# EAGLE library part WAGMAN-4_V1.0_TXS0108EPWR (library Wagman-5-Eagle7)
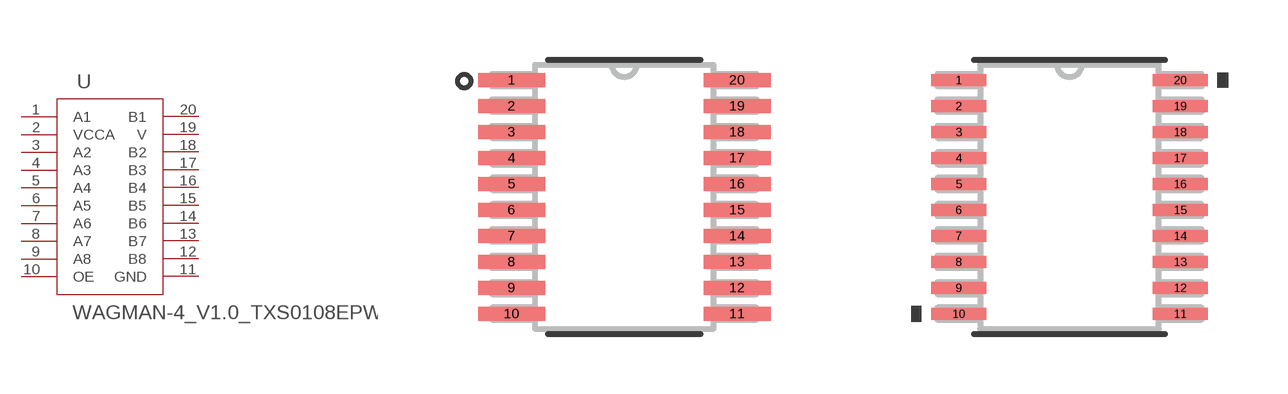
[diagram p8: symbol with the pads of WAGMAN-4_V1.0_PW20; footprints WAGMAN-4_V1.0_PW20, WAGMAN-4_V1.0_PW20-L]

Designator prefix U

## WAGMAN-4_V1.0_TXS0108EPWR (MANUFACTURER_PART_NUMBER: TXS0108EPWR; VENDOR: Texas Instruments)  [WAGMAN-4_V1.0_PW20]
1  A1
2  VCCA  pwr
3  A2
4  A3
5  A4
6  A5
7  A6
8  A7
9  A8
10  OE  out
11  GND  pwr
12  B8
13  B7
14  B6
15  B5
16  B4
17  B3
18  B2
19  V  pwr
20  B1

## WAGMAN-4_V1.0_TXS0108EPWRPW20-L (MANUFACTURER_PART_NUMBER: TXS0108EPWR; VENDOR: Texas Instruments)  [WAGMAN-4_V1.0_PW20-L]
Pads as for WAGMAN-4_V1.0_PW20

## WAGMAN-4_V1.0_TXS0108EPWRPW20-M (MANUFACTURER_PART_NUMBER: TXS0108EPWR; VENDOR: Texas Instruments)  [WAGMAN-4_V1.0_PW20-M]
Pads as for WAGMAN-4_V1.0_PW20

## Footprint WAGMAN-4_V1.0_PW20 (pad centres in mm)
smd 1.676 x 0.356: 1 -2.819,2.925; 2 -2.819,2.275; 3 -2.819,1.625; 4 -2.819,0.975; 5 -2.819,0.325; 6 -2.819,-0.325; 7 -2.819,-0.975; 8 -2.819,-1.625; 9 -2.819,-2.275; 10 -2.819,-2.925; 11 2.819,-2.925; 12 2.819,-2.275; 13 2.819,-1.625; 14 2.819,-0.975; 15 2.819,-0.325; 16 2.819,0.325; 17 2.819,0.975; 18 2.819,1.625; 19 2.819,2.275; 20 2.819,2.925

## Footprint WAGMAN-4_V1.0_PW20-L (pad centres in mm)
smd 1.372 x 0.305: 1 -2.769,2.925; 2 -2.769,2.275; 3 -2.769,1.625; 4 -2.769,0.975; 5 -2.769,0.325; 6 -2.769,-0.325; 7 -2.769,-0.975; 8 -2.769,-1.625; 9 -2.769,-2.275; 10 -2.769,-2.925; 11 2.769,-2.925; 12 2.769,-2.275; 13 2.769,-1.625; 14 2.769,-0.975; 15 2.769,-0.325; 16 2.769,0.325; 17 2.769,0.975; 18 2.769,1.625; 19 2.769,2.275; 20 2.769,2.925

## Footprint WAGMAN-4_V1.0_PW20-M (pad centres in mm)
smd 1.981 x 0.406: 1 -2.87,2.925; 2 -2.87,2.275; 3 -2.87,1.625; 4 -2.87,0.975; 5 -2.87,0.325; 6 -2.87,-0.325; 7 -2.87,-0.975; 8 -2.87,-1.625; 9 -2.87,-2.275; 10 -2.87,-2.925; 11 2.87,-2.925; 12 2.87,-2.275; 13 2.87,-1.625; 14 2.87,-0.975; 15 2.87,-0.325; 16 2.87,0.325; 17 2.87,0.975; 18 2.87,1.625; 19 2.87,2.275; 20 2.87,2.925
